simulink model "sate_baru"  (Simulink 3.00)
settings: Solver=ode45  StartTime=0.0  StopTime=100.0  RelTol=1e-3
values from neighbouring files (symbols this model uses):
  A = [0 1;-1/(L*C) -R/L]    [keadaan.m]    (also in optima1.m = [1 1 1 0 0 0 0; gudang.m = [1 0 1 0;0 1 0 1;-1 -1 -1 -1;1 1 0 0;0 0 1 1]; optima3.m = [1 1 1 0 0 0 0; optima2.m = [1 1 1 0 0 0 0)
  Am = A-B*K    [new_satelit_rev.m]
  B = [0;1/(L*C)]    [keadaan.m]    (also in optima1.m = [150 250 200 -500]; gudang.m = [150;75;-50;100;150]; optima3.m = [150 250 200 -500 -100 50]; optima2.m = [150 250 200 -500 b5x b6(i)])
  gam = 15    [new_satelit_rev.m]
  p3 = P(3,3)    [new_satelit_rev.m]
  p6 = P(3,2)    [new_satelit_rev.m]
  p7 = P(4,3)    [new_satelit_rev.m]
  p8 = P(3,1)    [new_satelit_rev.m]

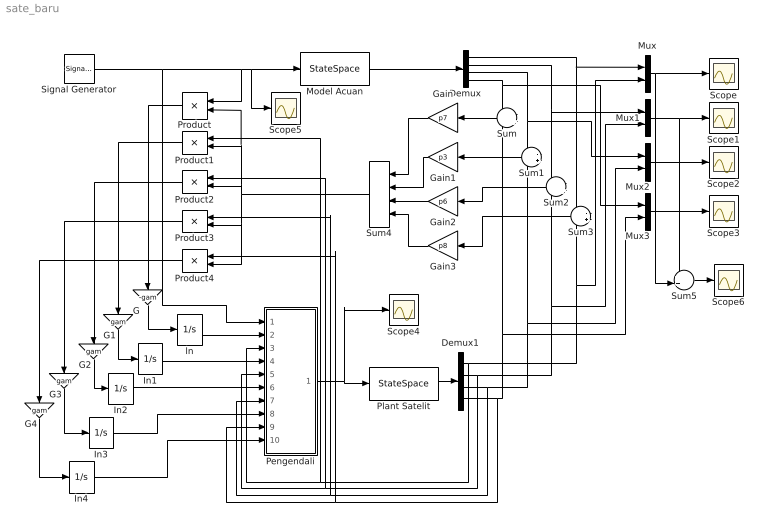
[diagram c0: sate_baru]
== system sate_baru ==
  Demux : Demux  Outputs=4
  Demux1 : Demux  Outputs=4
  G : Gain  Orientation=down  Gain=-gam  SaturateOnIntegerOverflow=on
  G{1..4} (4 alike) : Gain  Orientation=down  Gain=gam  SaturateOnIntegerOverflow=on
  Gain : Gain  Orientation=left  Gain=p7  SaturateOnIntegerOverflow=on
  Gain1 : Gain  Orientation=left  Gain=p3  SaturateOnIntegerOverflow=on
  Gain2 : Gain  Orientation=left  Gain=p6  SaturateOnIntegerOverflow=on
  Gain3 : Gain  Orientation=left  Gain=p8  SaturateOnIntegerOverflow=on
  In{1..4} (4 alike) : Integrator  ExternalReset=none  InitialConditionSource=internal  InitialCondition=0  LimitOutput=off  UpperSaturationLimit=inf  LowerSaturationLimit=-inf  ShowSaturationPort=off  ShowStatePort=off  AbsoluteTolerance=auto
  Model Acuan : StateSpace  A=Am  B=B  C=eye(4)  D=[0;0;0;0]  X0=[0;0;0;0]
  Mux{,1..3} (4 alike) : Mux  Inputs=2
  Pengendali : Subsystem
  Plant Satelit : StateSpace  A=A  B=B  C=eye(4)  D=[0;0;0;0]  X0=[0;0;0;0]
  Product{,1..4} (5 alike) : Product  Orientation=left  Inputs=2  SaturateOnIntegerOverflow=on
  Scope{,1..6} (7 alike) : Scope
  Signal Generator : SignalGenerator  WaveForm=square  Amplitude=0.1  Frequency=0.04  Units=Hertz
  Sum{,1..3} (4 alike) : Sum  Orientation=left  Inputs=-+
  Sum4 : Sum  Orientation=left  Inputs=++++
  Sum5 : Sum  Inputs=++|  SaturateOnIntegerOverflow=on
  ln : Integrator  ExternalReset=none  InitialConditionSource=internal  InitialCondition=0  LimitOutput=off  UpperSaturationLimit=inf  LowerSaturationLimit=-inf  ShowSaturationPort=off  ShowStatePort=off  AbsoluteTolerance=auto
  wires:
  Model Acuan/1 -> Demux/1
  Mux2/1 -> Scope2/1
  Mux3/1 -> Scope3/1
  Demux/1 -> Sum3/1, Mux/1
  Demux/4 -> Sum/1, Mux3/1
  Demux/2 -> Sum2/1, Mux1/1
  Demux/3 -> Sum1/1, Mux2/1
  G/1 -> ln/1
  G1/1 -> In1/1
  G2/1 -> In2/1
  G3/1 -> In3/1
  G4/1 -> In4/1
  Product/1 -> G/1
  Product1/1 -> G1/1
  Product2/1 -> G2/1
  Product3/1 -> G3/1
  Product4/1 -> G4/1
  Sum/1 -> Gain/1
  Sum1/1 -> Gain1/1
  Sum2/1 -> Gain2/1
  Sum3/1 -> Gain3/1
  Gain/1 -> Sum4/1
  Gain1/1 -> Sum4/2
  Gain2/1 -> Sum4/3
  Gain3/1 -> Sum4/4
  Signal Generator/1 -> Product/1, Model Acuan/1, Scope5/1, Pengendali/1(Uc)
  Sum4/1 -> Product/2, Product1/2, Product2/2, Product4/2, Product3/2
  Demux1/1 -> Pengendali/3(X1), Product1/1, Sum3/2, Mux/2
  Demux1/2 -> Pengendali/5(X2), Product2/1, Sum2/2, Mux1/2
  Demux1/3 -> Pengendali/7(X3), Product3/1, Sum1/2, Mux2/2
  ln/1 -> Pengendali/2(teta1)
  In1/1 -> Pengendali/4(teta2)
  In2/1 -> Pengendali/6(teta3)
  In3/1 -> Pengendali/8(teta4)
  In4/1 -> Pengendali/10(teta5)
  Pengendali/1(U) -> Plant Satelit/1, Scope4/1
  Demux1/4 -> Pengendali/9(X4), Product4/1, Sum/2, Mux3/2
  Plant Satelit/1 -> Demux1/1
  Mux1/1 -> Scope1/1, Sum5/1
  Mux/1 -> Scope/1, Sum5/2
  Sum5/1 -> Scope6/1

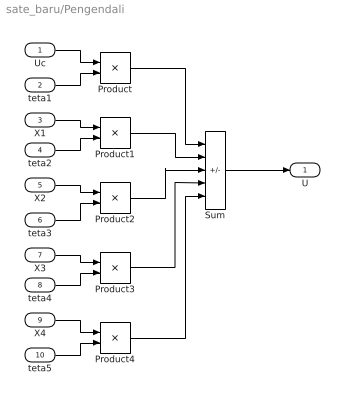
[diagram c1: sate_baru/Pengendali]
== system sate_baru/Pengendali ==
  Uc : Inport  Port=1  PortWidth=-1  SampleTime=-1  DataType=auto
  teta1 : Inport  Port=2  PortWidth=-1  SampleTime=-1  DataType=auto
  X1 : Inport  Port=3  PortWidth=-1  SampleTime=-1  DataType=auto
  teta2 : Inport  Port=4  PortWidth=-1  SampleTime=-1  DataType=auto
  X2 : Inport  Port=5  PortWidth=-1  SampleTime=-1  DataType=auto
  teta3 : Inport  Port=6  PortWidth=-1  SampleTime=-1  DataType=auto
  X3 : Inport  Port=7  PortWidth=-1  SampleTime=-1  DataType=auto
  teta4 : Inport  Port=8  PortWidth=-1  SampleTime=-1  DataType=auto
  X4 : Inport  Port=9  PortWidth=-1  SampleTime=-1  DataType=auto
  teta5 : Inport  Port=10  PortWidth=-1  SampleTime=-1  DataType=auto
  Product{,1..4} (5 alike) : Product  Inputs=2  SaturateOnIntegerOverflow=on
  Sum : Sum  Inputs=+----  SaturateOnIntegerOverflow=on
  U : Outport  Port=1
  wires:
  Sum/1 -> U/1
  Product/1 -> Sum/1
  Product1/1 -> Sum/2
  Product2/1 -> Sum/3
  Product3/1 -> Sum/4
  Product4/1 -> Sum/5
  Uc/1 -> Product/1
  teta1/1 -> Product/2
  X1/1 -> Product1/1
  teta2/1 -> Product1/2
  X2/1 -> Product2/1
  teta3/1 -> Product2/2
  X3/1 -> Product3/1
  teta4/1 -> Product3/2
  X4/1 -> Product4/1
  teta5/1 -> Product4/2
